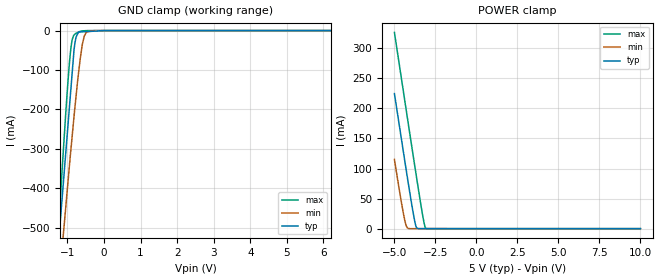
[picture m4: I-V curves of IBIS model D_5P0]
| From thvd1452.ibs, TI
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|   D_5p0 Model
[Model]   D_5P0
Model_type   Input
Vinl = 0.7
Vinh = 3.35
|   typ   min   max
C_comp   4.695pF   4.504pF   4.916pF
|  Where Nom  PVT is Nominal Process,   3.3V,  25C
|   Fast PVT is Strong Process,   3.6V, -40C
|   Slow PVT is Weak Process,   3V, 150C
[Model spec]
|subparameter
Vinl   0.462   0.420   0.504
Vinh   2.211   2.010   2.412
[Voltage Range]   5   4.5   5.5
|Junction Temperature
[Temperature Range]   25   150   -40
[Power Clamp Reference]   5   4.5   5.5
[GND Clamp Reference]   0   0   0
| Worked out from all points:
|   GND clamp passes 1 mA (typ) near -0.19 V on its own axis
|   POWER clamp passes 1 mA (typ) near -3.63 V on its own axis
[GND Clamp]
|   Voltage   I(typ)   I(min)   I(max)
-5V       -5.578A    -4.854A    -6.528A
-1.25V    -544.9mA   -660.5mA   -508.9mA
-1.141V   -419.4mA   -546.7mA   -345.5mA
-1.056V   -321.4mA   -458mA     -222.9mA
-991.4mV  -246.3mA   -389.9mA   -135.3mA
-905.3mV  -146.8mA   -301.1mA   -42.91mA
-819.4mV  -47.51mA   -216.6mA   -11.16mA
-790.6mV  -28.56mA   -189.8mA   -8.658mA
-642.3mV  -3.434mA   -65.57mA   -1.535mA
-539.2mV  -2.883mA   -13.61mA   -445uA
-274.1mV  -1.467mA   -25.44uA   -5.56uA
10V       0A         0A         0A
[POWER Clamp]
|   Voltage   I(typ)   I(min)   I(max)
-5V       224.6mA    115.1mA    326.4mA
-4.551V   145mA      40.18mA    245.7mA
-4.379V   114.6mA    15.3mA     214.9mA
-4.266V   94.83mA    3.843mA    194.5mA
-4.152V   75.1mA     313.8uA    174mA
-3.873V   28.68mA    17.01uA    124.3mA
-3.689V   4.175mA    15.82uA    91.91mA
-3.613V   505.7uA    15.33uA    78.66mA
-3.277V   23.7uA     13.15uA    22.02mA
-3.164V   22.37uA    12.42uA    6.07mA
-3.092V   21.53uA    11.95uA    735.4uA
10V       0A         0A         0A
